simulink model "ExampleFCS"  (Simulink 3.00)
settings: Solver=FixedStepDiscrete  StartTime=0.0  StopTime=10000.0  FixedStep=0.02  RelTol=1e-3
libraries: AVDSBlockset x1, simulink3 x1

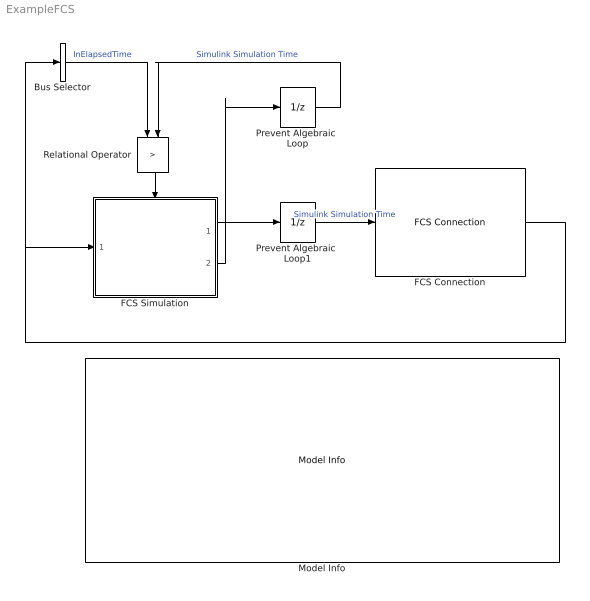
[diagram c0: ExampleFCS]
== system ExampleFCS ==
  Bus Selector : BusSelector  OutputSignals=InElapsedTime  MuxedOutput=off
  FCS Connection : AVDSBlockset/FCS Connection  Description=This block is used to connect Simulink to AVDS through the MATLAB AC model.
  FCS Simulation : Subsystem
  Model Info : simulink3/Signals & Systems/Model Info  InitialBlockCM=none  BlockCM=none  Frame=off  DisplayStringWithTags=|  HorizontalTextAlignment=Left  LeftAlignmentValue=0.02  SourceBlockDiagram=ExampleFCS  TagMaxNumber=20
      | Important -  make sure the files in the directory 
      |      "Utilities\MATLABToolbox\Toolbox\RequiredAVDSFiles" are installed
      |       according to the instructions in the file "ReadMe.RequiredAVDSFiles.txt".
      |    To start the simulation:
      |    1) Start AVDS
      |    2) Load the simulation initialization file "MATLAB_FCS.sim.ini". From the AVDS 
      |       menum, select "File->Simulation Init->Open" and choose the file 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
  Prevent Algebraic  Loop : UnitDelay  X0=0  SampleTime=0.02
  Prevent Algebraic  Loop1 : UnitDelay  X0=0  SampleTime=0.02
  Relational Operator : RelationalOperator  Orientation=down  Operator=>
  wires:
  Relational Operator/1 -> FCS Simulation/Enable
  Bus Selector/1 -> Relational Operator/1  "InElapsedTime"
  FCS Simulation/2(FCS Simulation Time) -> Prevent Algebraic  Loop/1
  Prevent Algebraic  Loop/1 -> Relational Operator/2  "Simulink Simulation Time"
  FCS Connection/1 -> Bus Selector/1, FCS Simulation/1(In1)
  FCS Simulation/1(Out To AVDS) -> Prevent Algebraic  Loop1/1
  Prevent Algebraic  Loop1/1 -> FCS Connection/1  "Simulink Simulation Time"

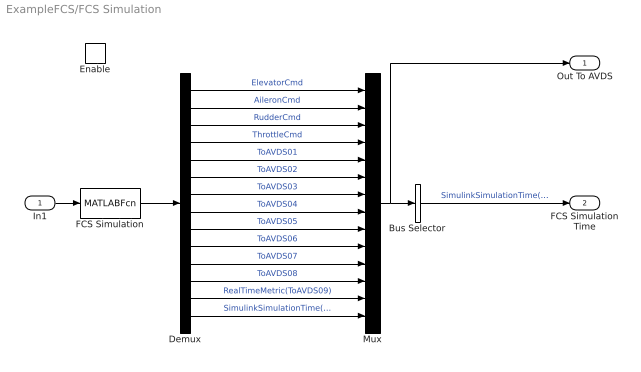
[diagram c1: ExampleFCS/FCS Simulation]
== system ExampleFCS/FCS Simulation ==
  In1 : Inport  Port=1  PortWidth=-1  SampleTime=-1  DataType=auto
  Enable : EnablePort
  Bus Selector : BusSelector  OutputSignals=SimulinkSimulationTime(ToAVDS10)  MuxedOutput=off
  Demux : Demux  Outputs=14
  FCS Simulation : MATLABFcn  MATLABFcn=AVDS_FCS_Simulink  OutputWidth=14  OutputSignalType=auto
  Mux : Mux  Inputs=14
  Out To AVDS : Outport  Port=1
  FCS Simulation Time : Outport  Port=2
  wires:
  Demux/1 -> Mux/1  "ElevatorCmd"
  Demux/2 -> Mux/2  "AileronCmd"
  Demux/3 -> Mux/3  "RudderCmd"
  Demux/4 -> Mux/4  "ThrottleCmd"
  Demux/5 -> Mux/5  "ToAVDS01"
  Demux/6 -> Mux/6  "ToAVDS02"
  Demux/7 -> Mux/7  "ToAVDS03"
  Demux/8 -> Mux/8  "ToAVDS04"
  Demux/9 -> Mux/9  "ToAVDS05"
  Demux/10 -> Mux/10  "ToAVDS06"
  Demux/11 -> Mux/11  "ToAVDS07"
  Demux/12 -> Mux/12  "ToAVDS08"
  Demux/13 -> Mux/13  "RealTimeMetric(ToAVDS09)"
  Demux/14 -> Mux/14  "SimulinkSimulationTime(ToAVDS10)"
  In1/1 -> FCS Simulation/1
  FCS Simulation/1 -> Demux/1
  Mux/1 -> Bus Selector/1, Out To AVDS/1
  Bus Selector/1 -> FCS Simulation Time/1  "SimulinkSimulationTime(ToAVDS10)"
